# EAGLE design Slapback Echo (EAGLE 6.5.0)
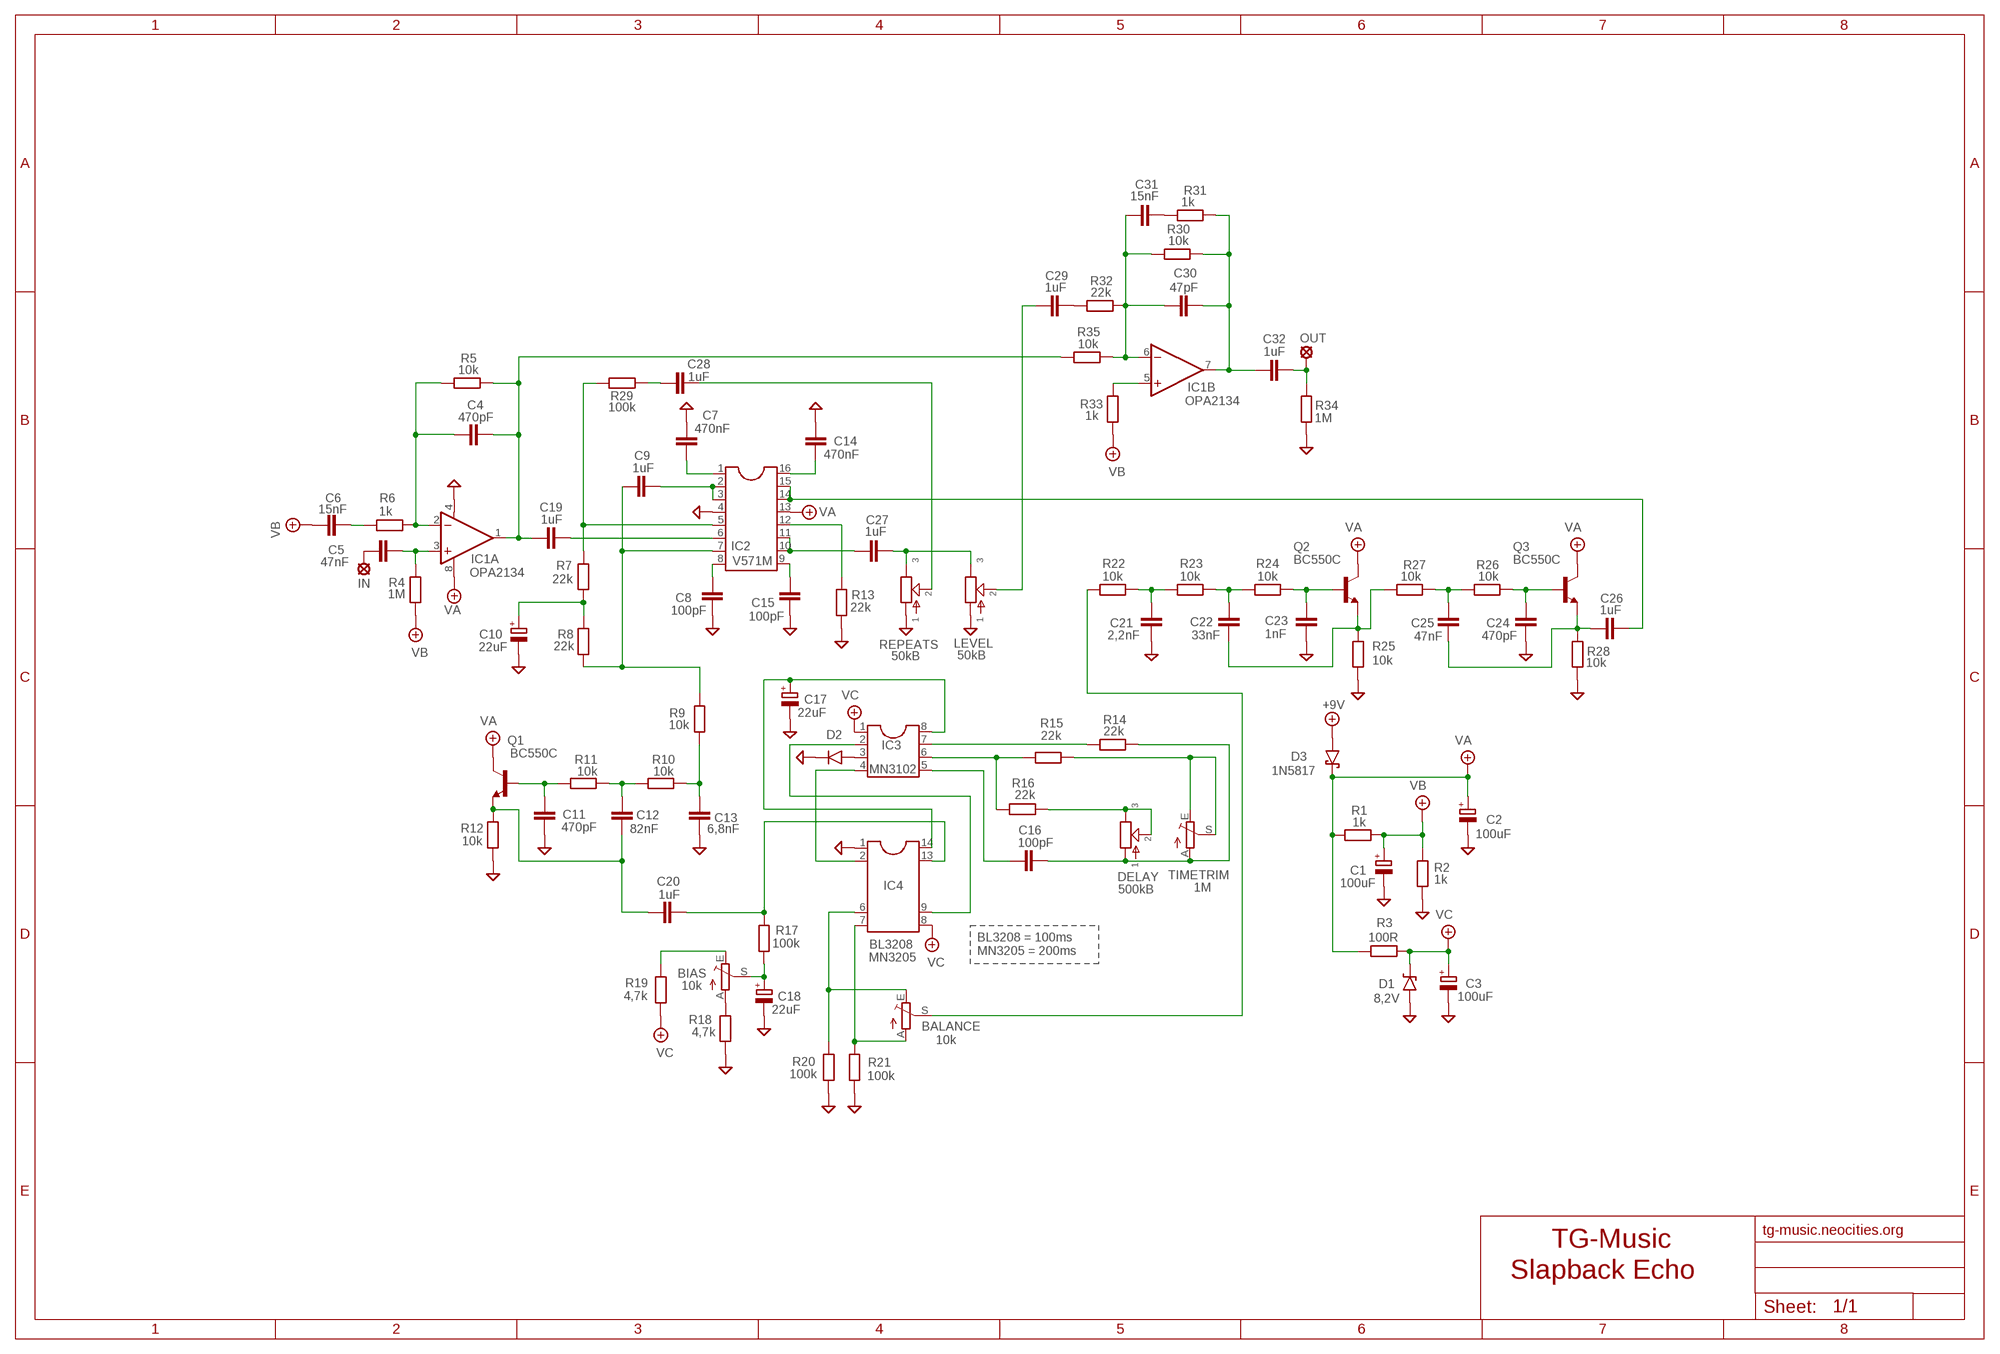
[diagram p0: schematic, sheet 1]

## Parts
+9V  +9V  +9V(T)1  [ROUND]
BALANCE  10k  TRIM_EU-PT10  [PT-10]
BIAS  10k  TRIM_EU-PT10  [PT-10]
C1  100uF  CPOL-EUD  [PANASONIC_D]
C2  100uF  CPOL-EUD  [PANASONIC_D]
C3  100uF  CPOL-EUD  [PANASONIC_D]
C4  470pF  050X030_0251  [050X030_025]
C5  47nF  22NF-82NF"  [4,5MM]
C6  15nF  1NF-15NF  [3,5MM]
C7  470nF  C-EUC0805  [C0805]
C8  100pF  C-EUC0805  [C0805]
C9  1uF  C-EUC0805  [C0805]
C10  22uF  CPOL-EUC  [PANASONIC_C]
C11  470pF  050X030_0251  [050X030_025]
C12  82nF  22NF-82NF"  [4,5MM]
C13  6,8nF  1NF-15NF  [3,5MM]
C14  470nF  C-EUC0805  [C0805]
C15  100pF  C-EUC0805  [C0805]
C16  100pF  050X030_0251  [050X030_025]
C17  22uF  CPOL-EUC  [PANASONIC_C]
C18  22uF  CPOL-EUC  [PANASONIC_C]
C19  1uF  072X0352  [072X035]
C20  1uF  072X0352  [072X035]
C21  2,2nF  1NF-15NF  [3,5MM]
C22  33nF  072X0252  [072X025]
C23  1nF  1NF-15NF  [3,5MM]
C24  470pF  050X030_0251  [050X030_025]
C25  47nF  072X0252  [072X025]
C26  1uF  072X0352  [072X035]
C27  1uF  072X0352  [072X035]
C28  1uF  072X0352  [072X035]
C29  1uF  072X0352  [072X035]
C30  47pF  050X030_0251  [050X030_025]
C31  15nF  1NF-15NF  [3,5MM]
C32  1uF  072X0352  [072X035]
D1  8,2V  1N9ZENER  [DO35-3]
D2  1N4148-3  [DO35-3]
D3  1N5817  [DO41-3]
DELAY  500kB  POT-EU16MM  [16MM]
GND  GND  GND(T)1  [ROUND]
GND1  GND  GND(T)1  [ROUND]
IC1  OPA2134  OPA2134P  [DIL08]
IC2  V571M  DIL16W  [SO16W]
IC3  MN3102  DIL8S  [SOCKET-08]
IC4  BL3208  DIL14/8  [DIL14/8]
IN  MCS10B  [MCS10B]
LEVEL  50kB  POT-EU16MM  [16MM]
OUT  MCS10B  [MCS10B]
Q1  BC550C  [TO92-EBC]
Q2  BC550C  [TO92-EBC]
Q3  BC550C  [TO92-EBC]
R1  1k  6MM-EU1  [R0207/1V]
R2  1k  6MM-EU1  [R0207/1V]
R3  100R  6MM-EU1  [R0207/1V]
R4  1M  6MM-EU1  [R0207/1V]
R5  10k  6MM-EU1  [R0207/1V]
R6  1k  6MM-EU1  [R0207/1V]
R7  22k  6MM-EU1  [R0207/1V]
R8  22k  6MM-EU1  [R0207/1V]
R9  10k  6MM-EU1  [R0207/1V]
R10  10k  6MM-EU1  [R0207/1V]
R11  10k  6MM-EU1  [R0207/1V]
R12  10k  6MM-EU1  [R0207/1V]
R13  22k  6MM-EU1  [R0207/1V]
R14  22k  6MM-EU1  [R0207/1V]
R15  22k  6MM-EU1  [R0207/1V]
R16  22k  6MM-EU1  [R0207/1V]
R17  100k  6MM-EU1  [R0207/1V]
R18  4,7k  6MM-EU1  [R0207/1V]
R19  4,7k  6MM-EU1  [R0207/1V]
R20  100k  6MM-EU1  [R0207/1V]
R21  100k  6MM-EU1  [R0207/1V]
R22  10k  6MM-EU1  [R0207/1V]
R23  10k  6MM-EU1  [R0207/1V]
R24  10k  6MM-EU1  [R0207/1V]
R25  10k  6MM-EU1  [R0207/1V]
R26  10k  6MM-EU1  [R0207/1V]
R27  10k  6MM-EU1  [R0207/1V]
R28  10k  6MM-EU1  [R0207/1V]
R29  100k  6MM-EU1  [R0207/1V]
R30  10k  6MM-EU1  [R0207/1V]
R31  1k  6MM-EU1  [R0207/1V]
R32  22k  6MM-EU1  [R0207/1V]
R33  1k  6MM-EU1  [R0207/1V]
R34  1M  6MM-EU1  [R0207/1V]
R35  10k  6MM-EU1  [R0207/1V]
REPEATS  50kB  POT-EU16MM  [16MM]
TIMETRIM  1M  TRIM_EU-PT10  [PT-10]

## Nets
+9V: +9V.1(+9V) D3.A
GND: C1.- C2.- C3.- C7.1 C8.1 C10.- C11.1 C13.2 C14.1 C15.1 C17.- C18.- C21.2 C23.2 C24.2 D1.A D2.C GND1.1(GND) GND.1(GND) IC1.4(A:V-) IC2.4 IC4.1 LEVEL.1 R2.1 R12.2 R13.1 R18.1 R20.1 R21.1 R25.1 R28.1 R34.1 REPEATS.1
N$1: C6.2 R6.1
N$2: C4.1 IC1.2(A:-IN) R5.1 R6.2
N$3: C5.2 IC1.3(A:+IN) R4.2
N$4: C4.2 C19.1 IC1.1(A:OUT) R5.2 R35.1
N$5: C5.1 IN.MP
N$6: C9.1 IC2.2 IC2.3
N$7: C7.2 IC2.1
N$8: BIAS.A R18.2
N$9: C9.2 IC2.7 R8.1 R9.2
N$10: C10.+ R7.1 R8.2
N$11: IC2.5 R7.2 R29.1
N$12: C12.2 C20.1 Q1.E R12.1
N$13: C11.2 Q1.B R11.2
N$14: C12.1 R10.2 R11.1
N$15: C13.1 R9.1 R10.1
N$16: C26.2 IC2.14 IC2.15
N$17: C15.2 IC2.9
N$18: C14.2 IC2.16
N$19: C8.2 IC2.8
N$20: IC2.12 R13.2
N$21: IC3.7 R14.2
N$22: IC3.6 R15.2 R16.2
N$23: C16.1 IC3.5
N$24: DELAY.2 DELAY.3 R16.1
N$25: R15.1 TIMETRIM.E TIMETRIM.S
N$26: C16.2 DELAY.1 R14.1 TIMETRIM.A
N$27: D2.A IC3.3
N$28: IC3.4 IC4.2
N$29: IC3.2 IC4.9
N$30: C17.+ IC3.8 IC4.14
N$31: C20.2 IC4.13 R17.2
N$32: BIAS.S C18.+ R17.1
N$34: BIAS.E R19.2
N$35: C27.1 IC2.10 IC2.11
N$36: BALANCE.A IC4.7 R21.2
N$37: BALANCE.E IC4.6 R20.2
N$38: C22.2 Q2.E R25.2 R27.1
N$39: C21.1 R22.2 R23.1
N$40: C22.1 R23.2 R24.1
N$41: C23.1 Q2.B R24.2
N$42: C25.1 R26.1 R27.2
N$43: C24.1 Q3.B R26.2
N$44: C25.2 C26.1 Q3.E R28.2
N$45: C27.2 LEVEL.3 REPEATS.3
N$46: BALANCE.S R22.1
N$47: C28.2 REPEATS.2
N$48: C29.2 R32.1
N$49: C28.1 R29.2
N$50: C29.1 LEVEL.2
N$51: C31.2 R31.1
N$52: C30.2 C32.1 IC1.7(B:OUT) R30.2 R31.2
N$53: IC1.5(B:+IN) R33.2
N$54: C30.1 C31.1 IC1.6(B:-IN) R30.1 R32.2 R35.2
N$55: C32.2 OUT.MP R34.2
N$56: C19.2 IC2.6
VA: C2.+ D3.C IC1.8(A:V+) IC2.13 Q1.C Q2.C Q3.C R1.1 R3.1
VB: C1.+ C6.1 R1.2 R2.2 R4.1 R33.1
VC: C3.+ D1.C IC3.1 IC4.8 R3.2 R19.1

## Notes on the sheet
- BL3208 = 100ms
  MN3205 = 200ms
- MN3205
- tg-music.neocities.org
- TG-Music

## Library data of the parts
+9V = Virransyöttö:+9V(T): +9V Voltage Supply
BALANCE BIAS TIMETRIM = pot:TRIM_EU-: POTENTIOMETER
C1-C3 C10 C17 C18 = rcl:CPOL-EU: POLARIZED CAPACITOR, European symbol
C4 C11 C16 C24 C30 = Keraamiset kondensaattorit:050X030_025: 47 - 120pF
C5 C12 = Mylar Kondensaattorit:22NF-82NF: 22nF-82nF
C6 C13 C21 C23 C31 = Mylar Kondensaattorit:1NF-15NF: 1nF-15nF
C7-C9 C14 C15 = rcl:C-EU: CAPACITOR, European symbol
C19 C20 C26-C29 C32 = Wima MKS:072X035: 0.15 - 1.0uF;
C22 C25 = Wima MKS:072X025: 1000pF - 0.47uF
D1 = Diodit:1N9*ZENER: 1N9???B Zener Diode
D2 = Diodit:1N4148: Fast Switching Diode
D3 = Diodit:1N5817
DELAY LEVEL REPEATS = potentiometers:POT-EU
GND GND1 = Virransyöttö:GND(T): Ground
IC1 = burr-brown:OPA2134: Operational Amplifier; MF: TEXAS INSTRUMENTS; MPN: OPA2134PA; OC_FARNELL: 1097574; OC_NEWARK: 74K3897
IC2 = ic-package:DIL16: Dual In Line / Socket
IC3 = ic-package:DIL8: Dual In Line / Socket
IC4 = ic-package:DIL14/8: Dual In Line
IN OUT = Padit:MCS10B: SOLDER PAD
Q1-Q3 = transistor-npn:BC550*: NPN Transistor
R1-R35 = gm-resistors:6MM-EU: 6mm Resistors (European schematic symbol)

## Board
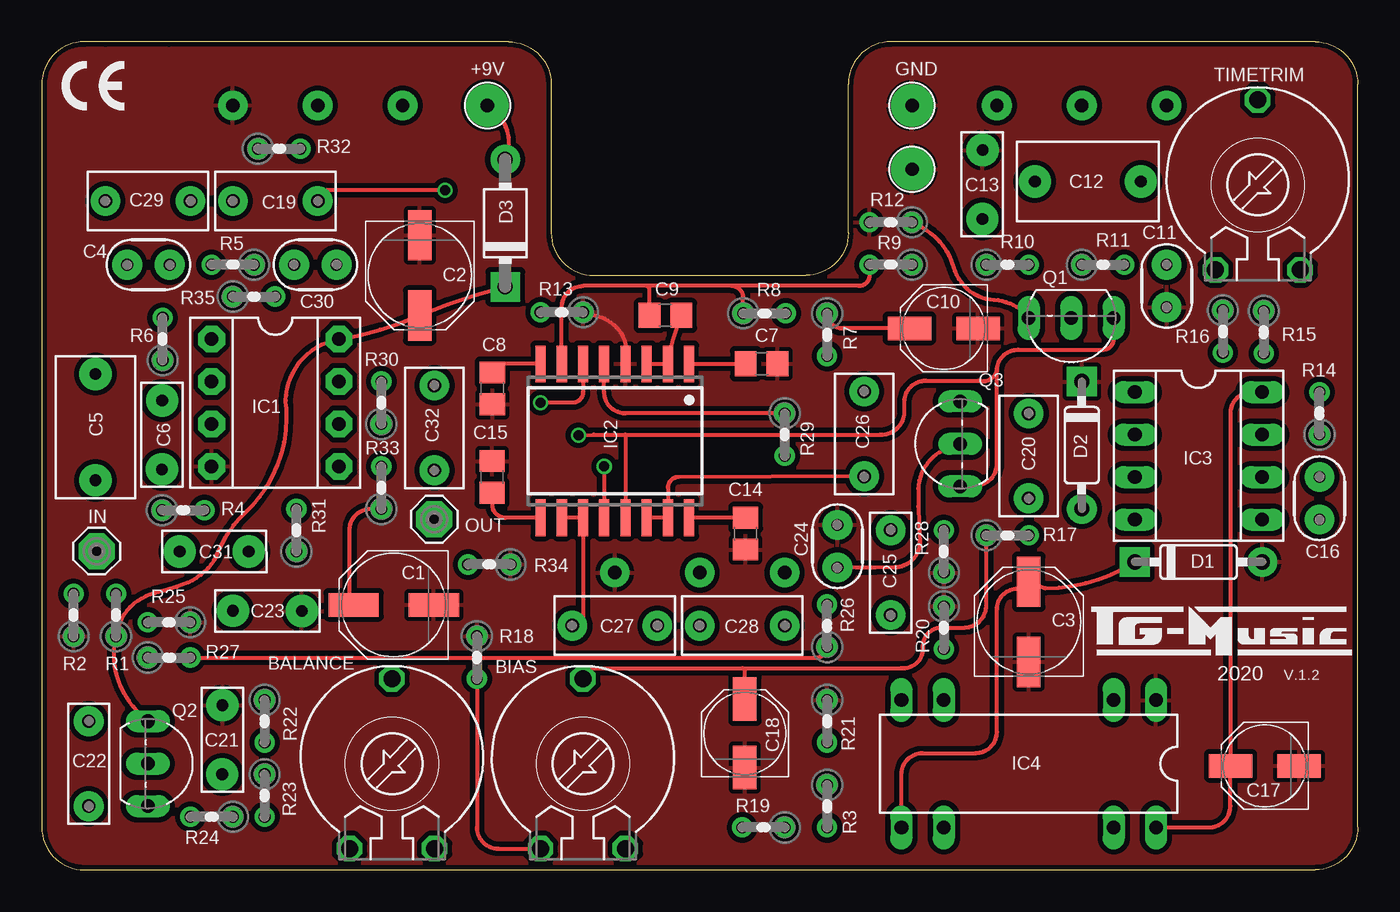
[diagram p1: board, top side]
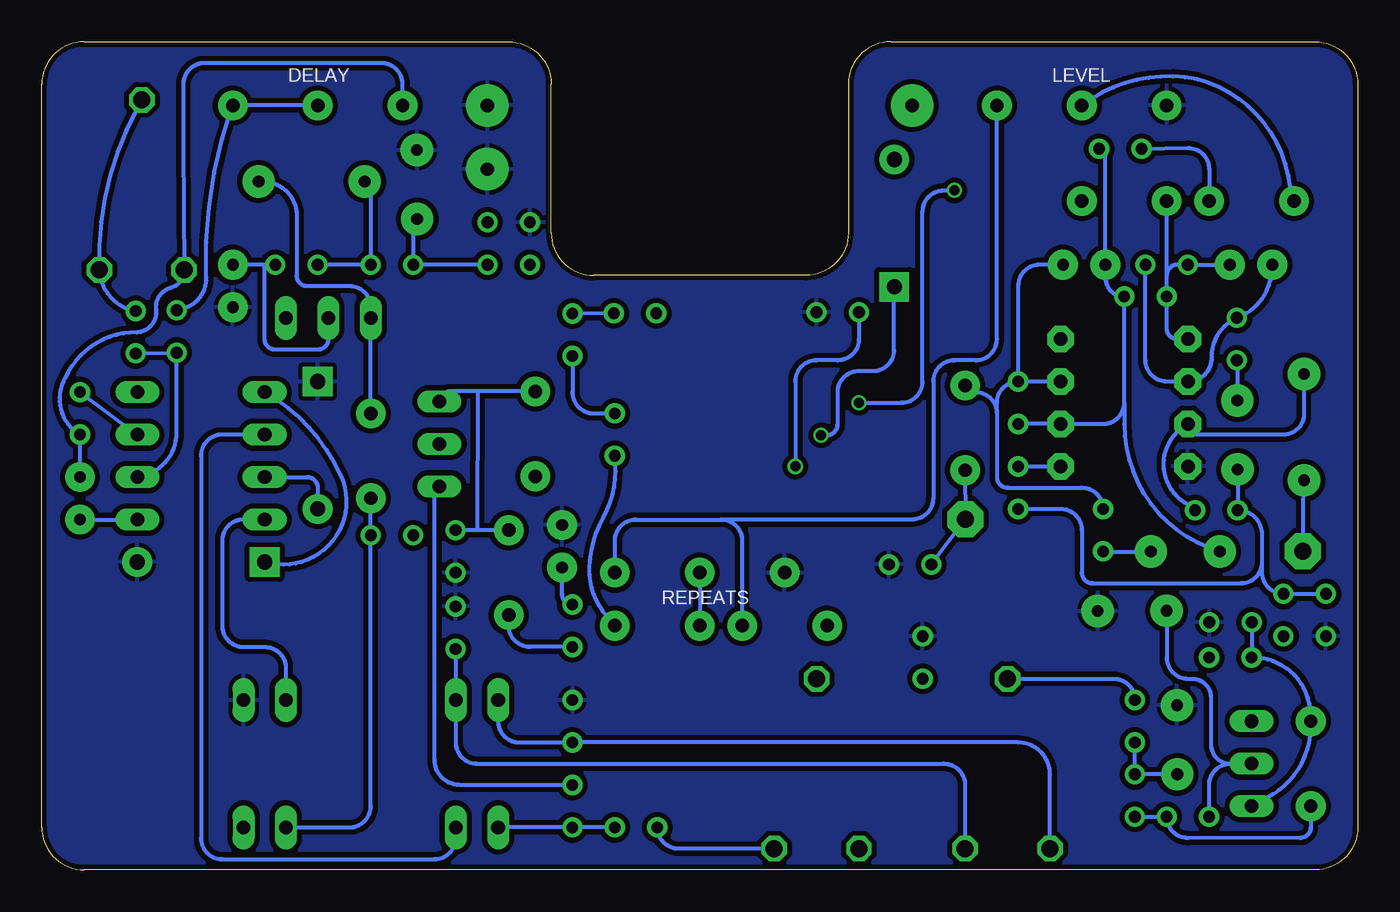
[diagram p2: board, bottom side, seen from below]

Size 78.74 x 49.53 mm. Coordinates in mm from the lower left corner, seen from the top.
Outline: 7.62,49.53 3.81,49.53
Outline: 78.74,2.54 78.74,46.99 arc90 76.2,49.53 50.8,49.53 arc90 48.26,46.99 48.26,38.1 arc-90 45.72,35.56 33.02,35.56 arc-90 30.48,38.1 30.48,46.99 arc90 27.94,49.53 2.54,49.53 arc90 0,46.99 0,2.54 arc90 2.54,0 76.2,0 arc90 78.74,2.54
Copper layers (1*16): Top 0.035mm / dielectric 1.5mm / Bottom 0.035mm
Design rules "ITEADstudio": minimum track width 10mil, minimum drill 12mil, track to track 12mil, track to pad 12mil, pad to pad 12mil, via to via 12mil, smd to smd 0mil, copper to edge 12mil, drill to drill 12mil, minimum pad ring 10mil, minimum via ring 6mil, stop-mask expansion 4mil, vias tented up to drill 100mil, thermal gap 10mil

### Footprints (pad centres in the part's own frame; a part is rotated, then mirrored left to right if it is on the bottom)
ROUND = drill 0.8 pad 2.54: 1 0,0
PT-10 = drill 1.016 octagon: A -2.54,-5.08; E 2.54,-5.08; S 0,5.08
PANASONIC_D = smd 3 x 1.4: + 2.4,0; - -2.4,0
050X030_025 = drill 0.7 pad 1.778: 1 -1.27,0; 2 1.27,0
4,5MM = drill 0.7 pad 1.93: 1 -3.175,0; 2 3.175,0
3,5MM = drill 0.7 pad 1.93: 1 -1.905,0; 2 2.221,-0.016
C0805 = smd 1.3 x 1.5: 1 -0.95,0; 2 0.95,0
PANASONIC_C = smd 2.6 x 1.4: + 2.05,0; - -2.05,0
072X035 = drill 0.8 pad 1.778: 1 -2.54,0; 2 2.54,0
072X025 = drill 0.8 pad 1.778: 1 -2.54,0; 2 2.54,0
DO35-3 = drill 0.9 pad 1.778: A 3.81,0 | drill 0.9 pad 1.778 square: C -3.81,0
DO41-3 = drill 0.9 pad 1.778: A 3.81,0 | drill 0.9 pad 1.778 square: C -3.81,0
16MM = drill 0.8 pad 1.778: 1 5.08,0; 2 0,0; 3 -5.08,0
DIL08 = drill 0.813 pad 1.6 octagon: 1 -3.81,-3.81; 2 -1.27,-3.81; 3 1.27,-3.81; 4 3.81,-3.81; 5 3.81,3.81; 6 1.27,3.81; 7 -1.27,3.81; 8 -3.81,3.81
SO16W = smd 0.6 x 2.2: 1 -4.445,-4.6; 2 -3.175,-4.6; 3 -1.905,-4.6; 4 -0.635,-4.6; 5 0.635,-4.6; 6 1.905,-4.6; 7 3.175,-4.6; 8 4.445,-4.6; 9 4.445,4.6; 10 3.175,4.6; 11 1.905,4.6; 12 0.635,4.6; 13 -0.635,4.6; 14 -1.905,4.6; 15 -3.175,4.6; 16 -4.445,4.6
SOCKET-08 = drill 0.813 long: 1 -3.81,-3.81; 2 -1.27,-3.81; 3 1.27,-3.81; 4 3.81,-3.81; 5 3.81,3.81; 6 1.27,3.81; 7 -1.27,3.81; 8 -3.81,3.81
DIL14/8 = drill 0.813 long: 1 -7.62,-3.81; 2 -5.08,-3.81; 6 5.08,-3.81; 7 7.62,-3.81; 8 7.62,3.81; 9 5.08,3.81; 13 -5.08,3.81; 14 -7.62,3.81
MCS10B = drill 1.016 pad 2.159 octagon: MP 0,0
TO92-EBC = drill 0.813 long: B 0,-1.27; C -2.54,-1.27; E 2.54,-1.27
R0207/1V = drill 0.7: 1 -1.27,0; 2 1.27,0

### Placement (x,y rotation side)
+9V  26.67,45.72 0 top
BALANCE  20.95,6.35 0 top
BIAS  32.38,6.35 0 top
C1  21.06,15.85 180 top
C2  22.62,35.56 270 top
C3  59.06,14.84 90 top
C4  6.39,36.19 0 top
C5  3.22,26.48 90 top
C6  7.19,25.86 90 top
C7  43.08,30.27 180 top
C8  26.96,28.8 90 top
C9  37.31,33.16 180 top
C10  53.98,32.38 180 top
C11  67.31,34.92 90 top
C12  62.59,41.17 0 top
C13  56.28,40.83 90 top
C14  42.12,20.11 90 top
C15  26.94,23.5 270 top
C16  76.45,22.23 90 top
C17  73.18,6.22 180 top
C18  42.07,8.17 90 top
C19  13.97,40.01 0 top
C20  59.05,24.77 270 top
C21  10.79,7.62 90 top
C22  2.81,6.35 90 top
C23  13.34,15.49 0 top
C24  47.61,19.36 90 top
C25  50.8,17.78 90 top
C26  49.21,26.08 270 top
C27  34.29,14.61 0 top
C28  41.91,14.61 180 top
C29  6.35,40.01 0 top
C30  16.37,36.2 0 top
C31  10.16,19.05 0 top
C32  23.5,26.44 270 top
D1  69.22,18.41 0 top
D2  62.23,25.4 270 top
D3  27.73,38.68 90 top
DELAY  62.23,45.72 0 bottom
GND  52.07,45.72 0 top
GND1  52.07,41.91 0 top
IC1  13.97,27.94 270 top
IC2  34.29,25.66 180 top
IC3  69.22,24.77 270 top
IC4  59.05,6.35 180 top
IN  3.29,19.07 0 top
LEVEL  16.51,45.72 0 bottom
OUT  23.49,20.98 0 top
Q1  61.59,31.75 180 top
Q2  7.62,6.35 270 top
Q3  53.67,25.48 90 top
R1  4.45,15.24 90 top
R2  1.91,15.24 90 top
R3  46.99,3.81 270 top
R4  8.46,21.51 0 top
R5  11.43,36.2 180 top
R6  7.23,31.75 90 top
R7  46.99,32.01 270 top
R8  43.24,33.29 0 top
R9  50.8,36.2 180 top
R10  57.78,36.2 0 top
R11  63.5,36.2 0 top
R12  50.8,38.73 180 top
R13  31.11,33.35 180 top
R14  76.45,27.3 90 top
R15  73.12,32.16 270 top
R16  70.67,32.2 270 top
R17  57.78,20.01 0 top
R18  26.04,12.7 270 top
R19  43.18,2.54 180 top
R20  53.98,14.48 270 top
R21  46.99,8.89 270 top
R22  13.34,8.89 270 top
R23  13.34,4.45 270 top
R24  10.16,3.17 180 top
R25  7.61,14.8 180 top
R26  46.99,14.61 90 top
R27  7.62,12.7 0 top
R28  53.98,19.05 90 top
R29  44.45,26.04 270 top
R30  20.32,27.94 90 top
R31  15.24,20.32 90 top
R32  14.21,43.14 0 top
R33  20.32,22.86 90 top
R34  26.78,18.27 180 top
R35  12.7,34.29 0 top
REPEATS  39.37,17.78 0 bottom
TIMETRIM  72.76,40.97 0 top

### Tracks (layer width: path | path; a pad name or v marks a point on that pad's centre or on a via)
+9V
  Top 0.254: +9V.1 27.1,45.34 arc-73 D3.A
GND
  Top 0.254: R13.1 33.29,33.11 arc-90 IC2.4
  pour Top: 0.09,2.2 0.09,47.08 arc-90 2.54,49.53 27.94,49.53 arc-90 30.48,46.99 30.48,38.1 arc90 33.02,35.56 45.72,35.56 arc90 48.26,38.1 48.26,46.99 arc-90 50.8,49.53 76.2,49.53 arc-90 78.74,46.99 78.74,2.54 arc-90 76.2,0 2.54,0 arc-90 0,2.54
  pour Bottom: 0,2.54 0,46.99 arc-90 2.54,49.53 27.94,49.53 arc-90 30.48,46.99 30.48,38.1 arc90 33.02,35.56 45.72,35.56 arc90 48.26,38.1 48.26,46.99 arc-90 50.8,49.53 76.2,49.53 arc-90 78.74,46.99 78.74,2.54 arc-90 76.2,0 2.54,0 arc-90
N$1
  Bottom 0.254: R6.1 7.2,30.48 C6.2
N$2
  Bottom 0.254: R5.1 12.7,30.48 arc-90 11.43,29.21 IC1.2 arc-91 8.73,30.67 arc67 R6.2 arc-71 C4.1
N$3
  Bottom 0.254: R4.2 10.13,21.81 arc-3 10.39,21.99 arc119 IC1.3 arc-90 9.53,26.04 4.45,26.04 arc-90 3.22,27.26 C5.2
N$4
  Bottom 0.254: C4.2 arc-90 C4.2 R5.2 10.79,36.2 arc-90 11.43,35.56 | IC1.1 10.79,31.75 arc90 11.43,32.38 R35.1 11.43,35.56 | 11.43,35.56 C19.1
N$5
  Bottom 0.254: IN.MP C5.1
N$6
  Top 0.254: IC2.3 IC2.2 arc-13 37.9,32.13 C9.1
N$7
  Top 0.254: IC2.1 42.11,30.26 arc90 C7.2
N$8
  Top 0.254: R18.2 26.04,2.54 arc90 27.3,1.27 BIAS.A
N$9
  Top 0.254: IC2.7 31.11,33.66 arc-90 32.38,34.92 36.2,34.92 | R8.1 41.97,34.23 arc90 41.27,34.92 | 41.27,34.92 36.2,34.92 | R9.2 49.53,35.56 arc-90 48.9,34.92 41.27,34.92 | C9.2 36.36,34.76 arc90 36.2,34.92
N$10
  Top 0.254: C10.+ 47.96,32.38 arc-90 R7.1
  Bottom 0.254: R8.2 R7.1
N$11
  Top 0.254: 33.66,30.48 IC2.5 33.66,28.57 arc90 34.92,27.3 R29.1
  Bottom 0.254: R7.2 46.99,28.57 arc-90 45.72,27.3 R29.1
N$12
  Top 0.254: R12.1 52.6,38.46 arc-46 54.55,36.05 arc71 56.99,34.1 arc-48 Q1.E
  Bottom 0.254: C20.1 Q1.E 59.05,33.66 arc-90 60.33,34.92 62.87,34.92 arc90 63.5,35.56 63.5,39.37 arc-90 C12.2
N$13
  Bottom 0.254: R11.2 65.41,36.2 | 65.41,36.2 C11.2 | Q1.B 61.59,31.75 arc90 62.23,31.11 64.77,31.11 arc90 65.41,31.75 65.41,36.2
N$14
  Bottom 0.254: R11.1 R10.2 59.05,41.17 C12.1
N$15
  Bottom 0.254: R9.1 R10.1 56.52,38.93 C13.1
N$16
  Top 0.254: IC2.14 IC2.15 37.47,22.86 arc-90 38.1,23.5 C26.2
N$17
  Top 0.254: IC2.9 27.75,21.06 arc-90 26.96,21.84 26.96,22.97 arc-90 C15.2
N$18
  Top 0.254: C14.2 arc90 C14.2 IC2.16
N$19
  Top 0.254: IC2.8 27.47,30.26 arc90 C8.2
N$20  (via drill 0.6)
  Top 0.254: v33.66,24.13 IC2.12
  Bottom 0.254: R13.2 29.84,31.75 arc90 31.11,30.48 32.38,30.48 arc-90 33.66,29.21 v33.66,24.13
N$21
  Bottom 0.254: R14.2 IC3.7
N$22
  Bottom 0.254: IC3.6 72.58,23.62 arc-75 70.67,26.15 arc1 R16.2 R15.2
N$23
  Bottom 0.254: C16.1 IC3.5
N$24
  Bottom 0.254: DELAY.2 DELAY.3 arc-22 68.89,35.44 arc77 70.28,33.58 R16.1
N$25
  Bottom 0.254: TIMETRIM.S 73.03,45.56 arc-31 TIMETRIM.E arc-78 R15.1
N$26
  Bottom 0.254: C16.2 R14.1 arc90 77.34,29.41 arc67 73.04,32.15 arc-95 71.91,33.5 arc82 71.04,34.81 arc-75 TIMETRIM.A arc1 70.27,46.98 arc90 68.99,48.26 58.42,48.26 arc90 57.15,46.99 DELAY.1
N$27
  Bottom 0.254: IC3.3 62.87,23.5 arc90 62.23,22.86 D2.A
N$28
  Bottom 0.254: IC3.4 66.67,20.95 arc-90 67.94,19.68 67.94,14.61 arc-90 66.67,13.34 65.41,13.34 arc90 64.14,12.06 IC4.2
N$29
  Bottom 0.254: IC3.2 67.94,26.04 arc-90 69.22,24.77 69.22,1.91 arc-90 67.94,0.64 55.24,0.64 arc-90 53.98,1.91 IC4.9
N$30
  Top 0.254: IC3.8 72.39,28.57 arc90 71.12,27.3 71.12,6.24 arc90 C17.+ arc90 C17.+ 71.12,3.81 arc-90 69.85,2.54 IC4.14
N$31
  Bottom 0.254: IC4.13 60.33,2.54 arc-90 59.05,3.81 R17.2 C20.2
N$32
  Top 0.254: 41.91,12.06 33.02,12.06 arc90 BIAS.S | 41.91,12.06 51.44,12.06 arc90 52.74,13.19 arc-90 53.68,14.49 55.24,14.49 arc90 56.52,15.88 R17.1 | C18.+ 42.06,11.91 arc90 41.91,12.06
N$34
  Bottom 0.254: BIAS.E 40.64,1.27 arc90 R19.2
N$35
  Top 0.254: IC2.10 IC2.11 32.38,15.24 arc-90 C27.1
N$36
  Bottom 0.254: IC4.7 51.44,8.89 arc-90 50.16,7.62 R21.2 20.32,7.62 arc90 18.41,5.71 BALANCE.A
N$37
  Bottom 0.254: R20.2 IC4.6 53.98,7.62 arc-90 52.7,6.35 24.77,6.35 arc90 23.5,5.08 BALANCE.E
N$38
  Bottom 0.254: R25.2 R27.1 arc90 2.82,9.32 C22.2 arc67 5.46,4.32 Q2.E
N$39
  Bottom 0.254: C21.1 R23.1 R22.2
N$40
  Bottom 0.254: C22.1 2.81,2.54 arc90 3.44,1.91 10.16,1.91 arc90 R24.1 R23.2
N$41
  Bottom 0.254: R24.2 8.89,5.08 arc90 7.62,6.35 | 7.62,6.35 Q2.B | C23.1 11.43,12.7 arc-90 10.16,11.43 9.91,11.43 arc90 8.79,10.31 8.79,7.52 arc-90 7.62,6.35
N$42
  Top 0.254: R27.2 46.35,12.7 arc90 R26.1
  Bottom 0.254: R26.1 49.53,13.34 arc90 50.8,14.61 C25.1
N$43
  Top 0.254: Q3.B 53.9,25.07 arc62 52.45,22.81 arc5 52.54,19.61 arc-89 51.02,18.09 arc-1 C24.1
  Bottom 0.254: R26.2 arc90 47.61,16.49 C24.1
N$44
  Bottom 0.254: C26.1 52.68,28.63 | 52.68,28.63 54.16,28.63 arc-90 Q3.E | C25.2 52.7,20.32 | 52.7,20.32 R28.2 | 52.68,28.63 52.7,20.32
N$45
  Bottom 0.254: REPEATS.3 44.45,19.68 arc90 43.18,20.95 38.1,20.95 | LEVEL.3 21.59,31.75 arc90 22.86,30.48 24.13,30.48 arc-90 25.4,29.21 25.4,22.23 arc90 26.67,20.95 38.1,20.95 | 38.1,20.95 arc90 36.83,19.68 C27.2
N$46
  Bottom 0.254: BALANCE.S 14.61,11.43 arc90 R22.1
N$47
  Bottom 0.254: REPEATS.2 C28.2
N$48
  Bottom 0.254: R32.1 10.16,43.18 arc90 8.89,41.91 C29.2
N$49
  Bottom 0.254: C28.1 44.95,15.19 arc42 45.97,18.02 arc28 45.13,21.1 arc-37 R29.2
N$50
  Bottom 0.254: C29.1 4.04,40.86 arc-69 9.6,47.28 arc-49 LEVEL.2
N$51
  Bottom 0.254: R31.1 arc-90 15.22,19.03 C31.2
N$52
  Bottom 0.254: IC1.7 R30.2 | C30.2 19.05,36.2 arc-90 20.32,34.92 R30.2 | 21.59,27.3 21.59,27.94 arc90 R30.2 | C32.1 22.86,28.57 arc90 21.59,27.3 | 21.59,27.3 21.59,23.5 arc-90 20.95,22.86 16.51,22.86 arc90 R31.2
N$53
  Bottom 0.254: R33.2 IC1.5
N$54
  Bottom 0.254: R30.1 IC1.6 15.24,26.67 arc-90 13.97,27.94 | 13.97,27.94 R35.2 arc90 15.1,35.42 C30.1 15.1,42.75 arc-90 R32.2 | 13.97,27.94 13.97,26.67 arc-74 C31.1
N$55
  Bottom 0.254: C32.2 OUT.MP R34.2
N$56  (via drill 0.6)
  Top 0.254: IC2.6 32.38,28.57 arc-90 31.75,27.94 v29.84,27.94 | v24.13,40.64 17.14,40.64 arc90 C19.2
  Bottom 0.254: v29.84,27.94 27.3,27.94 arc-90 26.04,29.21 26.04,39.37 arc90 24.77,40.64 v24.13,40.64
VA  (via drill 0.6)
  Top 0.254: 34.92,26.04 IC2.13 | Q3.C 55.91,23.02 arc90 57.15,24.26 57.15,29.84 | 57.15,29.84 arc-90 58.42,31.11 63.5,31.11 arc90 64.14,31.75 Q1.C | 34.92,26.04 50.16,26.04 arc90 51.62,27.36 51.62,27.99 arc-90 52.88,29.26 56.06,29.26 arc90 57.15,29.84 | Q2.C 5.78,9.44 arc-59 R1.1 arc-70 6.74,16.53 arc10 8.74,17.19 arc45 10.57,19.06 arc-26 12.09,21.28 arc52 14.61,27.71 arc-85 IC1.8 arc14 C2.+ arc-9 D3.C | v32.11,26 33.02,26.04 34.92,26.04
  Bottom 0.254: R3.1 53.73,5.08 arc90 55.23,6.58 55.23,22.65 arc90 Q3.C | v32.11,26 31.79,26 arc-90 31.11,26.67 31.11,28.57 arc90 29.84,29.84 28.99,29.84 arc-90 27.74,31.09 D3.C arc90 D3.C
VB
  Top 0.254: C1.+ 18.41,15.85 18.41,20.32 arc-90 19.68,21.59 R33.1
  Bottom 0.254: 5.71,18.41 arc90 6.99,17.14 15.88,17.14 arc90 16.51,17.78 16.51,20.32 arc-90 17.78,21.59 R33.1 | 5.71,18.41 5.71,20.04 arc-90 R4.1 arc-90 7.18,21.52 C6.1 | 5.71,18.41 5.71,17.78 arc-90 R1.2 R2.2
VC
  Top 0.254: D1.C arc-33 60.06,16.86 C3.+ arc-90 59.03,16.82 58.4,16.82 arc90 57.15,15.57 57.15,8.26 arc-90 55.88,6.99 52.7,6.99 arc90 51.44,5.71 IC4.8
  Bottom 0.254: R19.1 R3.2 IC4.8 | D1.C arc-131 60.85,23.6 arc-36 IC3.1

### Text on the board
tNames: 2020 | V.1.2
